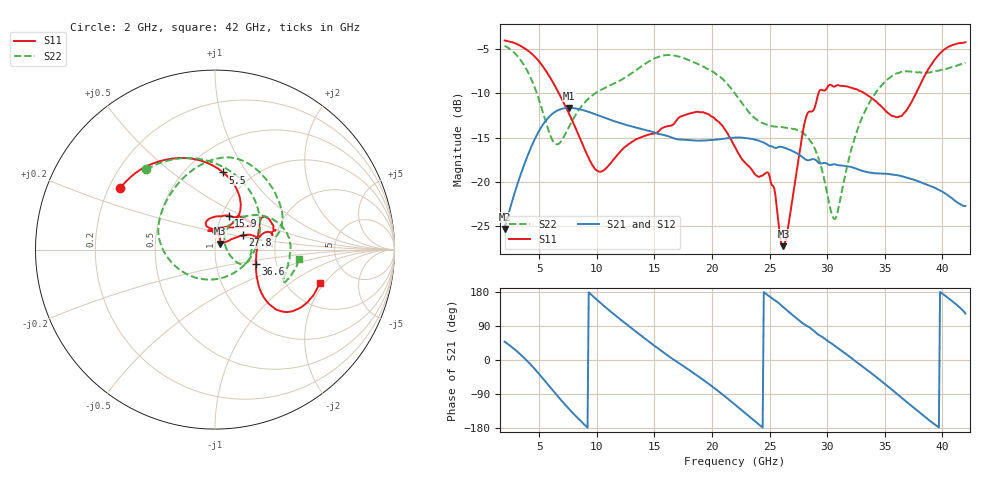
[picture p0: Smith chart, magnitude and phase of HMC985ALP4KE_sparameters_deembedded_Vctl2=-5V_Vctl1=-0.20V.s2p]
!s2p File: Measurements: S11, S21, S12, S22
# GHz S dB R 50.0
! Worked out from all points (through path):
!   401 points, 2 GHz to 42 GHz, reference 50 ohm
!   highest |S21| = -11.64 dB at 7.6 GHz (marker M1); lowest = -25.4 dB at 2 GHz (marker M2)
!   lowest |S11| = -27.3 dB at 26.2 GHz (marker M3), VSWR 1.09, Z = 52.8 + j3.48 ohm
!   |S11| at or under -10 dB: 6.717 GHz to 29.25 GHz (22.53 GHz wide, 125 % of centre); 33.26 GHz to 37.71 GHz (4.452 GHz wide, 12.5 % of centre)
!   |S22| runs from -24.2 to -4.6 dB; largest |S21 - S12| = 0.00025
!   S11 on the Smith chart (normalised r, x): 2 GHz: 0.25, +0.28; 5.5 GHz: 0.74, +0.78; 15.9 GHz: 1.08, +0.43; 27.8 GHz: 1.35, +0.22; 36.6 GHz: 1.56, -0.26; 42 GHz: 3.04, -1.81
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2  -4.01 147.1  -25.35 48.4  -25.36 48.4  -4.61 130.6
3.6  -4.79 120.4  -18.43 8.2  -18.43 8.2  -6.64 85.2
5.5  -7.29 83.9  -13.22 -55.2  -13.22 -55.2  -12.89 2.2
6.5  -9.46 66.9  -12.00 -91.6  -12.00 -91.6  -15.77 -70.3
7.6  -12.32 55.9  -11.64 -129.5  -11.65 -129.5  -13.76 -136.8
8.7  -15.57 57.6  -11.86 -163.9  -11.86 -163.9  -11.42 -170.9
10.2  -18.86 86.4  -12.52 153.9  -12.52 153.9  -9.72 164.7
11.9  -16.81 110.1  -13.31 110.6  -13.32 110.6  -8.64 141.4
15.4  -14.25 76.3  -14.61 28.8  -14.61 28.9  -5.85 87.3
15.9  -13.80 67.9  -14.74 17.7  -14.74 17.7  -5.68 81.1
19.4  -12.22 34.2  -15.34 -55.9  -15.34 -55.9  -7.08 35.6
22  -16.07 51.9  -15.00 -117.9  -15.01 -117.9  -10.01 10.4
24.9  -19.00 103.5  -15.89 169.6  -15.89 169.6  -13.61 13.1
26.2  -27.30 49.8  -16.11 139.2  -16.12 139.2  -13.84 -1.6
27.8  -15.08 27.0  -17.16 98.7  -17.16 98.8  -14.38 -22.8
28.7  -12.03 12.7  -17.45 80.6  -17.45 80.6  -15.66 -29.3
30.7  -9.20 20.7  -18.04 36.4  -18.04 36.4  -24.21 22.8
32.9  -9.75 33.9  -18.71 -13.5  -18.72 -13.5  -13.15 52.4
35.4  -12.33 11.3  -19.14 -72.6  -19.14 -72.6  -8.28 21.9
36.6  -12.34 -19.3  -19.43 -103.0  -19.43 -103.0  -7.56 6.7
39.6  -5.78 -42.3  -20.86 -175.9  -20.85 -175.9  -7.46 -25.0
42  -4.22 -17.5  -22.75 122.5  -22.76 122.5  -6.52 -6.2
